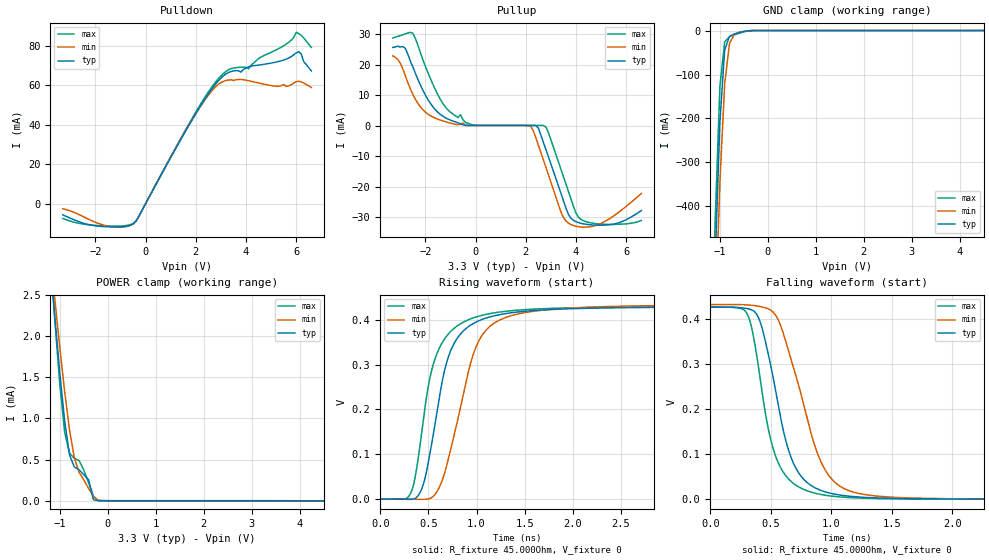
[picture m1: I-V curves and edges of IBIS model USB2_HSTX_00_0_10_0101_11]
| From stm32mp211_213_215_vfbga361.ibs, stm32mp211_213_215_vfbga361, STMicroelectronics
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[Model] USB2_HSTX_00_0_10_0101_11
Model_type   Output
Polarity   Non-Inverting
Enable   Active-High
C_comp   8.036pF   7.631pF   8.569pF
Vmeas = 200.000mV
Vref = 200.000mV
Rref = 45Ohms
Cref = 0pF
[Model Spec]
Vmeas   200.000mV   200.000mV   200.000mV
Vref   200.000mV   200.000mV   200.000mV
| This model is not intended for timing simulations.
| Warnings about Cref, Vref & Rref can be ignored
[Temperature Range]   25.000   125.000   -40.000
[Voltage Range]   3.300V   3.070V   3.630V
[GND Clamp Reference]   0.00V   0.00V   0.00V
[Pulldown Reference]   0.00V   0.00V   0.00V
[POWER Clamp Reference]   3.300V   3.070V   3.630V
[Pullup Reference]   3.300V   3.070V   3.630V
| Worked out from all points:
|   slope of the pulldown table from 0 to 0.495 V, typ, clamps not added: 42.6 ohm
|   GND clamp passes 1 mA (typ) near -0.43 V on its own axis
|   POWER clamp passes 1 mA (typ) near -0.91 V on its own axis
|   rising waveform, R_fixture 45.000Ohm, V_fixture 0: 20-80 % time 253ps typ, 307ps min, 236ps max; typ from 0 V to 0.428 V
|   falling waveform, R_fixture 45.000Ohm, V_fixture 0: 20-80 % time 215ps typ, 280ps min, 184ps max; typ from 0.427 V to 0 V
[GND Clamp]
-3.3V     -11.02A    -10.62A    -11.32A
-1.2V     -931.6mA   -1.049A    -855.7mA
-1.1V     -533.1mA   -671.7mA   -440.2mA
-1V       -209.4mA   -347mA     -127.3mA
-900mV    -44.44mA   -121.7mA   -25.6mA
-800mV    -13.15mA   -29.48mA   -14.15mA
-700mV    -7.743mA   -9.125mA   -9.769mA
-500mV    -2.127mA   -1.981mA   -2.894mA
-300mV    -19.53uA   -62.22uA   -13.79uA
6.6V      10.37uA    26.59uA    21.05uA
[Power Clamp]
-3.3V     3.206A     2.175A     4.855A
-1.2V     2.88mA     3.008mA    2.969mA
-1.1V     2.195mA    2.419mA    2.156mA
-1V       1.545mA    1.852mA    1.406mA
-900mV    967.9uA    1.324mA    831.4uA
-800mV    558.5uA    864.6uA    580.3uA
-700mV    412uA      525.9uA    517uA
-600mV    376.6uA    345uA      488.5uA
-400mV    254.2uA    146.6uA    216.8uA
-300mV    11.21uA    52.87uA    53.51uA
-100mV    94.86nA    985nA      361.1nA
6.6V      -2.695uA   -5.181uA   -2.897uA
[Pulldown]
-3.3V     -5.671mA   -2.581mA   -7.449mA
-1.6V     -11.64mA   -11.09mA   -11.31mA
-500mV    -10.25mA   -10.32mA   -10.1mA
1.9V      43.42mA    43.46mA    44.13mA
2.9V      62.15mA    60.37mA    63.26mA
3.4V      66.87mA    62.63mA    68.29mA
4.1V      69.19mA    62.19mA    68.26mA
4.5V      70.11mA    61.06mA    73.4mA
5.6V      73.12mA    59.29mA    80.76mA
6V        76.33mA    61.79mA    86.69mA
6.1V      76.89mA    61.93mA    85.99mA
6.6V      67.17mA    58.79mA    79.1mA
[Pullup]
-3.3V     25.59mA    22.83mA    28.68mA
-2.8V     25.32mA    16.37mA    30mA
-2.5V     19.22mA    10.28mA    30.28mA
-1.7V     6.185mA    2.827mA    13.54mA
-400mV    111.7uA    77.66uA    1.021mA
2.2V      68.65uA    -248.8uA   104.8uA
2.5V      -771uA     -6.355mA   83.49uA
2.8V      -7.784mA   -13.58mA   -409.8uA
3.4V      -22.12mA   -28.2mA    -14.26mA
3.8V      -30.28mA   -32.32mA   -24mA
4.4V      -32.24mA   -33.17mA   -31.39mA
6.6V      -27.75mA   -22.18mA   -30.98mA
[Ramp]
R_load=45.000Ohm
dV/dt_r   628.635mV/1.060ns  596.904mV/1.085ns  682.277mV/1000.000ps
dV/dt_f   630.819mV/240.000ps  599.810mV/315.000ps  684.093mV/215.000ps
[Rising waveform]
R_fixture=45.000Ohm
V_fixture=0
0s        451.9nV    3.128uV    468nV
330ps     -314.7uV   -409.1uV   20.78mV
450ps     34.97mV    -426uV     181mV
590ps     195.4mV    17.05mV    325.2mV
670ps     288.9mV    59.67mV    357.8mV
770ps     348.3mV    145.3mV    381.2mV
960ps     390.6mV    318.7mV    403.6mV
1.12ns    404.9mV    381.4mV    412.8mV
2.39ns    426.3mV    429.4mV    427.4mV
9.9ns     427.9mV    433.8mV    427.8mV
[Falling waveform]
R_fixture=45.000Ohm
V_fixture=0
0s        427.4mV    433.2mV    427.3mV
310ps     423.7mV    432.1mV    409.5mV
410ps     396.3mV    428.9mV    273mV
540ps     241.6mV    409.4mV    95.75mV
620ps     134.7mV    354.7mV    53.86mV
700ps     73.01mV    281.9mV    32.88mV
950ps     16.59mV    64.99mV    9.138mV
1.17ns    6.372mV    17.19mV    3.608mV
1.69ns    1.254mV    2.767mV    886uV
9.9ns     14.1uV     30.45uV    4.715uV
